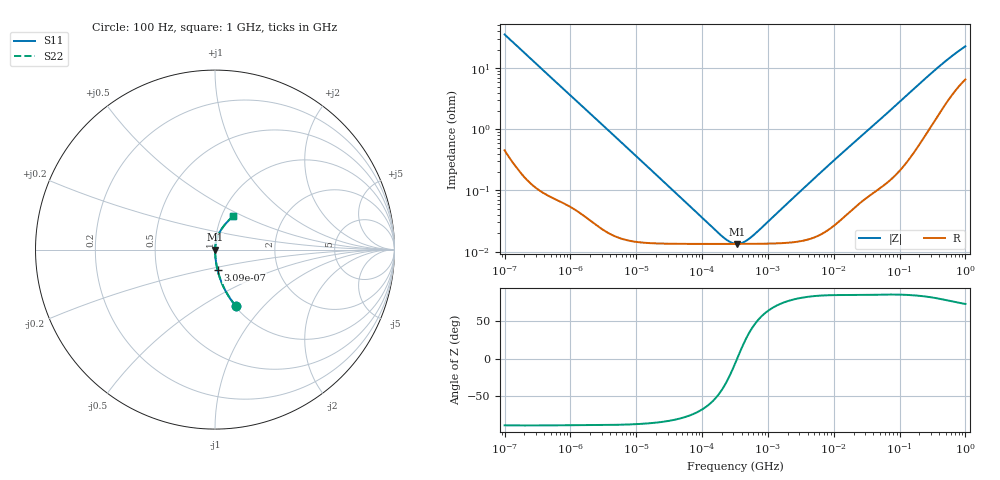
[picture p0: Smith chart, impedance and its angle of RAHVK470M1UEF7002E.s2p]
! RAHVK470M1UEF7002E  S-PARAMETER MODEL  (AEC-Q200 qualified)
! Model Generated by ELNA Corporation (http://www.ty-top.com)
! Version 1.0
! ELNA Control No. 201214
! Copyright (c) 2020 ELNA CO.,LTD. All Rights Reserved.
! Products Name : CONDUCTIVE POLYMER HYBRID ALUMINUM ELECTROLYTIC CAPACITORS
! Characteristics :
!  Capacitance  :  47uF  ,  Rated voltage  :  50V
!  Operating Temp. Range  :  -55 to +125 degC  ,  Endurance  :  4000hr at 125 degC
!  Dimension D  :  8mm  ,  Dimension L  :  8.7mm
! Frequency Range : 100Hz - 1GHz
! External Node Assignments :
!  1  o---| |---o  2
# MHz S RI R 50
!Freq[MHz].  S11 Real  S11 Imag  S21 Real  S21 Imag  S12 Real  S12 Imag  S22 Real  S22 Imag
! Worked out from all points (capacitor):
!   401 points, 100 Hz to 1 GHz, reference 50 ohm
!   read as one part in series: C = 44.7 uF near 108 Hz
!   lowest |Z| = 13.4 mohm at 342.8 kHz (marker M1)
!   series resonance near 341 kHz, so ESL is about 4.9 nH
!   S11 on the Smith chart (normalised r, x): 100 Hz: 1.01, -0.71; 309 Hz: 1.00, -0.23; 1 GHz: 1.13, +0.44
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0.0001  0.1157 -0.3135  0.8843 0.3135  0.8843 0.3135  0.1157 -0.3135
0.000113  0.0933 -0.2851  0.9067 0.2851  0.9067 0.2851  0.0933 -0.2851
0.000162  0.0479 -0.2087  0.9521 0.2087  0.9521 0.2087  0.0479 -0.2087
0.000309  0.0142 -0.1136  0.9858 0.1136  0.9858 0.1136  0.0142 -0.1136
0.000613  0.00408 -0.058  0.9959 0.058  0.9959 0.058  0.00408 -0.058
0.001488  0.000993 -0.0242  0.999 0.0242  0.999 0.0242  0.000993 -0.0242
0.004241  0.000262 -0.00856  0.9997 0.00856  0.9997 0.00856  0.000262 -0.00856
0.022131  0.000138 -0.00164  0.9999 0.00164  0.9999 0.00164  0.000138 -0.00164
0.187284  0.000134 -0.000136  0.9999 0.000136  0.9999 0.000136  0.000134 -0.000136
0.248313  0.000134 -6.88e-05  0.9999 6.88e-05  0.9999 6.88e-05  0.000134 -6.88e-05
0.316228  0.000134 -1.61e-05  0.9999 1.61e-05  0.9999 1.61e-05  0.000134 -1.61e-05
0.342768  0.000134 1.12e-06  0.9999 -1.12e-06  0.9999 -1.12e-06  0.000134 1.12e-06
0.386812  0.000134 2.7e-05  0.9999 -2.7e-05  0.9999 -2.7e-05  0.000134 2.7e-05
0.436516  0.000134 5.32e-05  0.9999 -5.32e-05  0.9999 -5.32e-05  0.000134 5.32e-05
0.578762  0.000134 0.000118  0.9999 -0.000118  0.9999 -0.000118  0.000134 0.000118
4.704354  0.000168 0.00146  0.9998 -0.00146  0.9998 -0.00146  0.000168 0.00146
12.37371  0.000333 0.00378  0.9997 -0.00378  0.9997 -0.00378  0.000333 0.00378
69.9842  0.00182 0.0197  0.9982 -0.0197  0.9982 -0.0197  0.00182 0.0197
176.8072  0.00697 0.0484  0.993 -0.0484  0.993 -0.0484  0.00697 0.0484
380.1894  0.0259 0.0966  0.9741 -0.0966  0.9741 -0.0966  0.0259 0.0966
668.3439  0.0613 0.1465  0.9387 -0.1465  0.9387 -0.1465  0.0613 0.1465
1000  0.0993 0.1849  0.9007 -0.1849  0.9007 -0.1849  0.0993 0.1849
